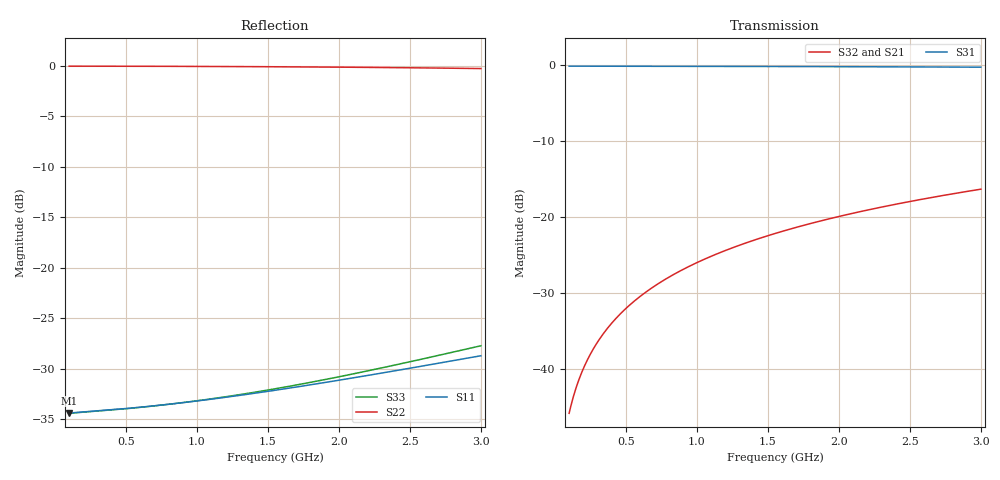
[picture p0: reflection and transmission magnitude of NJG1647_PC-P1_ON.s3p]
! NJG1647HD3 S-parameter(touchstone)
! 1bit SPDT switch with D/D converter
! Port1=P1, Port2=P2, Port3=PC
! VDD=2.7V, VCTL=1.8V, PC-P1 ON, D/D con ON
# hz S ma R 50
! freq  magS11  angS11  magS12  angS12  magS13  angS13
!  magS21  angS21
!  magS22  angS22  magS23  angS23
!  magS31  angS31  magS32  angS32
!  magS33  angS33
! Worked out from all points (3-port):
!   291 points, 100 MHz to 3 GHz, reference 50 ohm
!   strongest paths, dB at 100 MHz, 820 MHz, 1.55 GHz, 2.28 GHz, 3 GHz:
!     S31: -0.2, -0.2, -0.2, -0.3, -0.3
!     S32: -45.8, -27.8, -22.2, -18.8, -16.4
!     S21: -46.2, -28.1, -22.5, -19.1, -16.6
!   lowest |S11| = -34.4 dB at 100 MHz (marker M1), VSWR 1.04, Z = 51.9 - j0.143 ohm
!   |S11| at or under -10 dB: start of sweep to end of sweep
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1e8  0.01903 -4.2  0.004923 76.9  0.9787 -1.0
     0.004923 76.9  0.9971 -1.6  0.005106 76.9
     0.9787 -1.0  0.005106 76.9  0.01897 -4.8
1.7e8  0.01919 -7.0  0.008245 80.7  0.9785 -1.7
       0.008245 80.7  0.9971 -2.6  0.00855 80.8
       0.9785 -1.7  0.00855 80.8  0.01914 -8.1
2.6e8  0.0194 -10.6  0.01255 81.9  0.9784 -2.7
       0.01255 81.9  0.997 -4.0  0.01302 82.0
       0.9784 -2.7  0.01302 82.0  0.01935 -12.2
3.8e8  0.0197 -15.3  0.01832 81.7  0.9781 -3.9
       0.01832 81.7  0.9968 -5.9  0.01899 81.9
       0.9781 -3.9  0.01899 81.9  0.01965 -17.7
5.3e8  0.02012 -21.2  0.02554 80.5  0.9778 -5.4
       0.02554 80.5  0.9964 -8.2  0.02647 80.8
       0.9778 -5.4  0.02647 80.8  0.02008 -24.5
7.2e8  0.02074 -28.4  0.0347 78.5  0.9773 -7.4
       0.0347 78.5  0.9958 -11.2  0.03597 78.9
       0.9773 -7.4  0.03597 78.9  0.02072 -32.9
9.5e8  0.02163 -36.9  0.04583 75.7  0.9765 -9.7
       0.04583 75.7  0.9947 -14.8  0.04749 76.3
       0.9765 -9.7  0.04749 76.3  0.02166 -42.8
1.55e9  0.02468 -57.5  0.07508 67.9  0.9741 -15.9
        0.07508 67.9  0.9905 -24.2  0.07769 68.9
        0.9741 -15.9  0.07769 68.9  0.02509 -67.4
2.2e9  0.02921 -77.6  0.1072 59.0  0.9703 -22.6
       0.1072 59.0  0.9835 -34.6  0.1108 60.4
       0.9703 -22.6  0.1108 60.4  0.03077 -91.3
3e9  0.0366 -99.5  0.1476 47.8  0.9638 -30.8
     0.1476 47.8  0.9704 -47.8  0.152 49.7
     0.9638 -30.8  0.152 49.7  0.04101 -116.5
